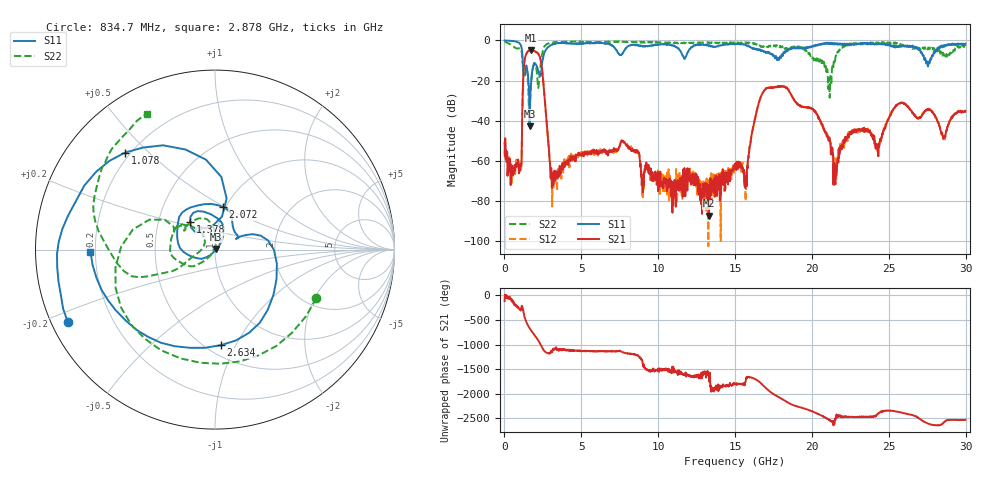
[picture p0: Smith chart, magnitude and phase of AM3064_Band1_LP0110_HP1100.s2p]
# Hz S DB R 50.0
!freq dBS11 angS11 dBS21 angS21 dBS12 angS12 dBS22 angS22
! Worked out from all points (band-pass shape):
!   1600 points, 10 MHz to 29.98 GHz, reference 50 ohm
!   highest |S21| = -4.76 dB at 1.716 GHz (marker M1); lowest = -87.2 dB at 13.28 GHz (marker M2)
!   |S21| within 3 dB of the highest: 1.369 GHz to 2.281 GHz (912.1 MHz wide, 50 % of centre)
!   lowest |S11| = -42.7 dB at 1.641 GHz (marker M3), VSWR 1.01, Z = 50.6 + j0.361 ohm
!   |S11| at or under -10 dB: 1.186 GHz to 2.476 GHz (1.29 GHz wide, 70.4 % of centre); 27.4 GHz to 27.68 GHz (282.9 MHz wide, 1.03 % of centre)
!   |S22| runs from -42.5 to -0.4 dB; largest |S21 - S12| = 0.0074
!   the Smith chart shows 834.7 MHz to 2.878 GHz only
!   S11 on the Smith chart (normalised r, x): 834.7 MHz: 0.05, -0.23; 1.078 GHz: 0.18, +0.42; 1.378 GHz: 0.72, +0.23; 2.072 GHz: 0.97, +0.49; 2.634 GHz: 0.59, -0.87; 2.878 GHz: 0.18, -0.01
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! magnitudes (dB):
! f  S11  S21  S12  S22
! 10 MHz  0.0  -50.9  -54.9  -0.4
! 834.7 MHz  -0.8  -61.8  -63.3  -4.1
! 1.078 GHz  -2.6  -62.6  -63.4  -4.5
! 1.378 GHz  -13.7  -7.5  -7.5  -13.7
! 1.641 GHz  -42.7  -4.9  -4.8  -35.6
! 1.716 GHz  -22.5  -4.8  -4.8  -23.1
! 2.072 GHz  -12.3  -5.8  -5.8  -13.6
! 2.634 GHz  -5.5  -30.6  -30.5  -2.7
! 2.878 GHz  -3.2  -52.6  -53.9  -1.5
! 3.178 GHz  -1.9  -72.0  -73.3  -1.2
! 5.015 GHz  -1.5  -57.4  -56.3  -0.7
! 7.714 GHz  -6.3  -50.5  -50.2  -0.7
! 10 GHz  -2.0  -75.0  -74.8  -1.0
! 13.28 GHz  -2.9  -87.2  -68.5  -1.2
! 15 GHz  -1.9  -64.0  -63.8  -1.4
! 15.68 GHz  -2.4  -71.9  -79.8  -1.2
! 17.03 GHz  -6.0  -23.7  -23.7  -3.5
! 19.99 GHz  -3.4  -33.9  -34.0  -8.2
! 21.13 GHz  -1.2  -48.2  -50.4  -21.2
! 21.55 GHz  -1.7  -62.4  -66.8  -7.7
! 25 GHz  -2.0  -38.6  -38.8  -1.2
! 29.98 GHz  -1.7  -35.1  -35.3  -2.8
